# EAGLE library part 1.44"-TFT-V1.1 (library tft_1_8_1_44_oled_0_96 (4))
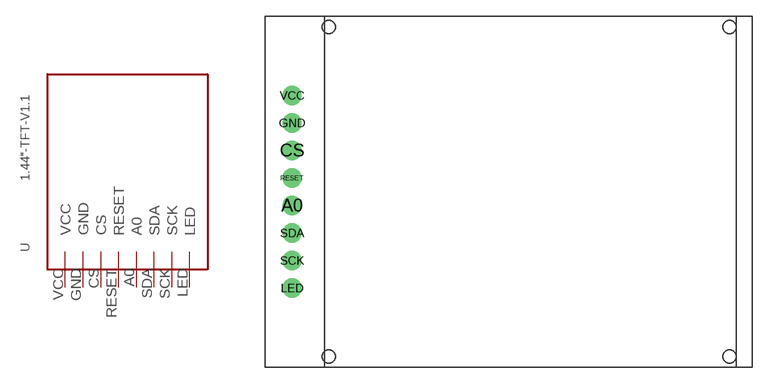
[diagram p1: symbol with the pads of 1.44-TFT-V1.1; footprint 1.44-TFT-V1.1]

Designator prefix -

## 1.44"-TFT-V1.1  [1.44-TFT-V1.1]
A0  A0
CS  CS
GND  GND
LED  LED
RESET  RESET
SCK  SCK
SDA  SDA
VCC  VCC

## Footprint 1.44-TFT-V1.1 (pad centres in mm)
drill 1 pad 1.778: A0 0,7.62; CS 0,12.7; GND 0,15.24; LED 0,0; RESET 0,10.16; SCK 0,2.54; SDA 0,5.08; VCC 0,17.78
